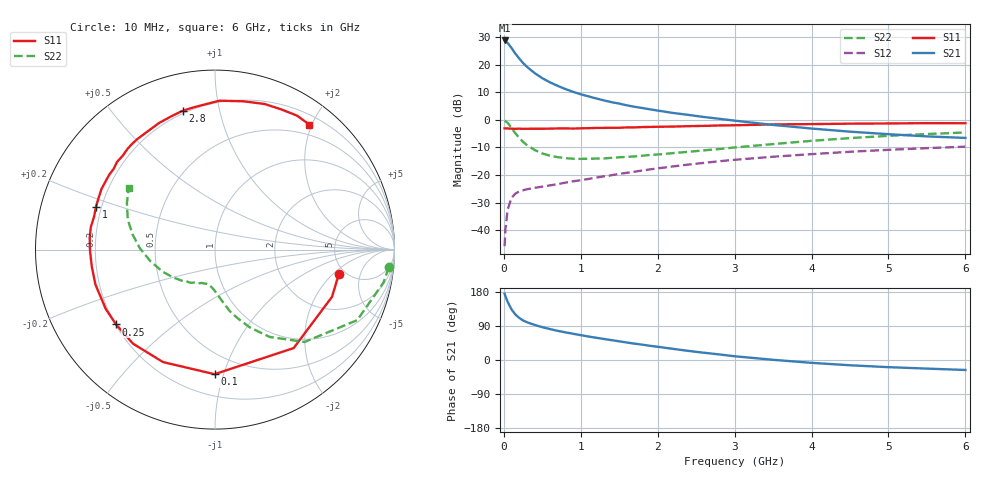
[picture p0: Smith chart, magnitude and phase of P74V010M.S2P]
! SIEMENS Small Signal Semiconductors
! BFP196
! Si NPN RF Bipolar Junction Transistor in SOT143
! VCE = 4 V  IC = 10 mA
! Common Emitter S-Parameters:  May  1996
# GHz  S  MA  R  50
!  f  S11  S21  S12  S22
! GHz  MAG  ANG  MAG  ANG  MAG  ANG  MAG  ANG
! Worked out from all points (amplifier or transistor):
!   36 points, 10 MHz to 6 GHz, reference 50 ohm
!   highest |S21| = 28.9 dB at 10 MHz (marker M1)
!   |S21| within 3 dB of that: start of sweep to 106.4 MHz
!   unconditionally stable (mu >= 1): 883.1 MHz to 3.267 GHz
!   at 250 MHz: K = 0.40, MSG = 23.1 dB, |S12| = -25.5 dB
!   at 1.4 GHz: K = 1.14, MAG = 11.0 dB, |S12| = -20.1 dB
!   at 6 GHz: K = 0.97, MSG = 1.6 dB, |S12| = -9.7 dB
!   S11 on the Smith chart (normalised r, x): 10 MHz: 4.38, -2.39; 100 MHz: 0.35, -0.93; 250 MHz: 0.20, -0.32; 1 GHz: 0.18, +0.17; 2.8 GHz: 0.19, +0.78; 6 GHz: 0.34, +1.96
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0.01  0.7033 -11.3  27.82 175.1  0.0051 86.2  0.9738 -5.8
0.02  0.703 -22.0  27.02 168.3  0.0102 81.0  0.9564 -11.1
0.05  0.7022 -51.4  25.01 153.2  0.0238 66.7  0.8844 -26.4
0.1  0.6941 -90.2  20.3 133.4  0.0385 51.2  0.7167 -45.9
0.15  0.6903 -114.8  16.02 120.0  0.0459 42.1  0.5726 -58.1
0.2  0.6952 -131.1  13.08 111.1  0.0505 37.1  0.4733 -66.0
0.25  0.691 -142.9  10.84 104.4  0.0528 34.3  0.399 -72.1
0.3  0.6926 -151.6  9.237 99.7  0.0551 33.3  0.3512 -76.6
0.4  0.694 -163.8  7.121 92.6  0.0586 32.7  0.2851 -82.6
0.5  0.693 -172.2  5.737 86.6  0.0615 33.4  0.2466 -87.4
0.6  0.6964 -179.5  4.824 81.6  0.0648 35.1  0.2242 -91.5
0.7  0.7014 174.5  4.166 76.9  0.0683 36.6  0.2111 -95.0
0.8  0.7031 169.7  3.647 73.0  0.0727 37.8  0.2027 -98.2
1  0.7051 160.1  2.931 65.6  0.0806 40.4  0.1964 -103.4
1.1  0.7095 156.1  2.682 62.0  0.0848 41.7  0.1975 -106.2
1.6  0.7325 138.2  1.842 46.1  0.1099 43.8  0.2135 -119.9
2.2  0.7583 119.5  1.34 29.4  0.1433 42.3  0.2501 -135.1
2.8  0.7944 103.1  1.051 14.7  0.1779 37.8  0.297 -152.1
3.5  0.83 88.3  0.813 0.5  0.2149 30.6  0.3648 -169.6
4.5  0.8571 71.2  0.613 -13.9  0.2646 19.8  0.4682 169.4
5.5  0.8753 58.5  0.503 -22.7  0.3078 8.4  0.5554 152.1
6  0.8726 52.9  0.472 -26.3  0.3273 2.2  0.5922 144.3
